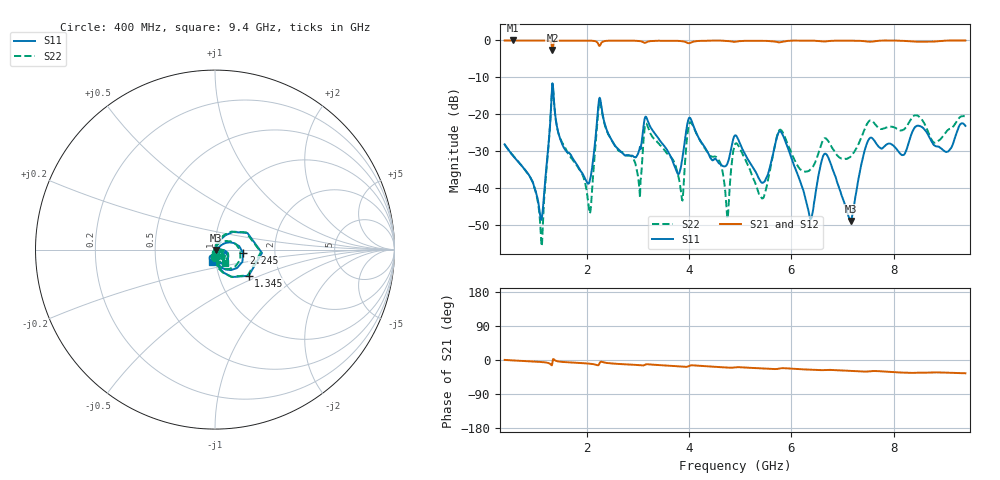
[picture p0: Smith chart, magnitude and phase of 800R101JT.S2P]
!  American Technical Ceramics  Date:  6/19/09
!  One Norden Lane
!  Huntington Station,  NY.  11746-2102
!  Tel:  (631) 622-4700  Fax:  (631) 622-4748
!  Part Number  800R101JT
!  Description: Ultra-low ESR, NPO  Mounting Orientation: Horizontal
!  Application: High RF power Filters, Combiners, Matching networks,
!  Antenna, DC block, Bypass and Couplers
# GHZ S DB R 50
! Freq  |S11|  S11 Ph  |S21|  S21 Ph  |S12|  S12 Ph  |S22|  S22 Ph
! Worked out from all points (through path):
!   801 points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, 400 MHz to 9.4 GHz, reference 50 ohm
!   highest |S21| = 0.00 dB at 569 MHz (marker M1); lowest = -2.6 dB at 1.334 GHz (marker M2)
!   group delay of S21, straight-line fit = 10.7 ps
!   lowest |S11| = -49.0 dB at 7.161 GHz (marker M3), VSWR 1.01, Z = 50.3 - j0.208 ohm
!   |S11| at or under -10 dB: start of sweep to end of sweep
!   |S22| runs from -55.8 to -11.8 dB; largest |S21 - S12| = 0.0035
!   S11 on the Smith chart (normalised r, x): 400 MHz: 1.00, -0.08; 1.345 GHz: 1.38, -0.43; 2.245 GHz: 1.37, -0.06; 9.4 GHz: 0.95, -0.13
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0.4  -28.19 -89.0  -0.01 0.3  -0.02 0.3  -28.18 -89.6
0.569  -31.37 -89.5  0.00 -1.2  -0.02 -1.2  -31.29 -91.7
1.12  -48.66 -6.6  -0.01 -5.4  -0.03 -5.4  -55.81 -172.2
1.334  -11.62 -4.1  -2.61 -7.4  -2.62 -7.3  -11.83 -3.1
1.345  -12.49 -38.0  -1.85 2.3  -1.86 2.3  -12.67 -38.0
1.908  -35.81 -66.8  -0.03 -8.2  -0.04 -8.1  -36.11 -116.8
2.076  -37.28 3.7  -0.05 -9.9  -0.07 -9.9  -46.44 140.7
2.245  -16.01 -7.1  -1.42 -11.5  -1.43 -11.5  -16.96 -2.8
3.021  -30.06 -16.4  -0.14 -13.6  -0.15 -13.6  -38.61 -129.5
3.404  -26.55 -89.8  -0.08 -13.2  -0.09 -13.2  -27.92 -111.2
3.854  -33.56 -13.1  -0.18 -17.1  -0.19 -17.1  -42.12 -84.2
4.056  -21.93 -66.7  -0.47 -14.0  -0.48 -13.9  -22.55 -79.1
4.743  -33.65 -35.8  -0.11 -19.9  -0.12 -19.8  -47.08 -103.5
4.9  -25.76 -47.3  -0.37 -19.3  -0.38 -19.3  -28.18 -54.0
5.429  -38.61 -46.8  -0.10 -22.1  -0.10 -22.1  -42.89 -53.5
5.8  -24.82 -57.9  -0.43 -21.8  -0.44 -21.8  -24.31 -50.7
6.408  -47.25 -25.0  -0.06 -25.9  -0.06 -25.8  -34.49 -28.9
6.666  -30.73 -51.2  -0.26 -26.2  -0.26 -26.1  -26.51 -40.1
7.161  -48.97 -35.6  -0.04 -28.7  -0.03 -28.7  -31.47 -20.9
7.499  -27.20 -25.9  -0.32 -30.3  -0.32 -30.2  -22.21 -19.1
7.904  -27.97 -82.5  -0.01 -31.3  -0.01 -31.2  -23.45 -47.3
9.4  -23.17 -106.0  -0.01 -35.0  -0.01 -34.9  -20.59 -51.6
